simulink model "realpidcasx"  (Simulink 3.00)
settings: Solver=ode45  SolverMode=SingleTasking  StartTime=0.0  StopTime=50  FixedStep=st_size  MaxStep=st_size  RelTol=1e-5  AbsTol=1e-6
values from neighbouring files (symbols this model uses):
  Disturb = Setpoint    [mimo_MSF1DF_sim.m]    (also in mimo_MSF2DF_sim.m)
  K = 1/kpd    [imc2pseucon.m]    (also in imc2pseudo.m)
  Satlb = temp1    [cback.m]    (also in imcmenu.m = str2num(satlbs))
  Satub = temp1    [cback.m]    (also in imcmenu.m = str2num(satubs))
  Setpoint = zeros(1,n)    [mimo_MSF1DF_sim.m]    (also in mimo_MSF2DF_sim.m)
undefined symbols (not defined in the file or in its folder): conv, denCs2, K1, numCs2, Qdden, TauD, TauD1, TauI, TauI1, XdenPs, XnumPs, Xpdeadx

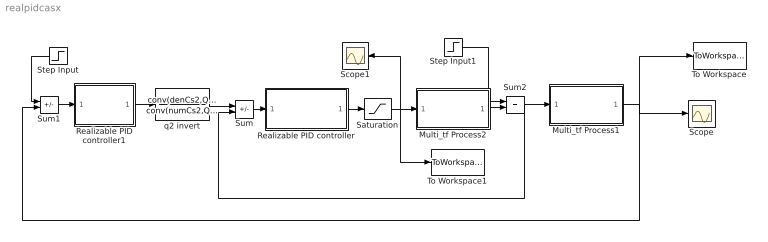
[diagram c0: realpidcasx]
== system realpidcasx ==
  Multi_tf Process1 : Subsystem
  Multi_tf Process2 : Subsystem
  Realizable PID controller : Subsystem
  Realizable PID controller1 : Subsystem
  Saturation : Saturate  UpperLimit=Satub  LowerLimit=Satlb
  Scope : Scope
  Scope1 : Scope
  Step Input : Step  Orientation=left  Time=0  Before=0  After=Setpoint  SampleTime=0
  Step Input1 : Step  Time=0  Before=0  After=Disturb  SampleTime=0
  Sum : Sum  Inputs=+-  SaturateOnIntegerOverflow=on
  Sum1 : Sum  Inputs=+-  SaturateOnIntegerOverflow=on
  Sum2 : Sum  Inputs=++  SaturateOnIntegerOverflow=on
  To Workspace : ToWorkspace  VariableName=simout  SampleTime=-1  SaveFormat=Matrix
  To Workspace1 : ToWorkspace  VariableName=effort  SampleTime=-1  SaveFormat=Matrix
  q2 invert : TransferFcn  Numerator=conv(denCs2,Qdden)  Denominator=conv(numCs2,Qdden)
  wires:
  Sum/1 -> Realizable PID controller/1(In1)
  Multi_tf Process2/1(Out1) -> Sum2/2
  Step Input1/1 -> Sum2/1
  Realizable PID controller/1(Out1) -> Saturation/1
  Saturation/1 -> To Workspace1/1, Multi_tf Process2/1(In1), Scope1/1
  Sum2/1 -> Sum/2, Multi_tf Process1/1(In1)
  Step Input/1 -> Sum1/1
  Realizable PID controller1/1(Out1) -> q2 invert/1
  Sum1/1 -> Realizable PID controller1/1(In1)
  q2 invert/1 -> Sum/1
  Multi_tf Process1/1(Out1) -> Sum1/2, To Workspace/1, Scope/1

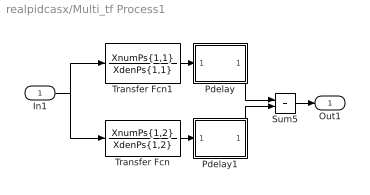
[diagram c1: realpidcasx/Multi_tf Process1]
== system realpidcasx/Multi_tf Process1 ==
  In1 : Inport  Port=1  PortWidth=-1  SampleTime=-1  DataType=auto
  Pdelay : Subsystem
  Pdelay1 : Subsystem
  Sum5 : Sum  Inputs=++  SaturateOnIntegerOverflow=on
  Transfer Fcn : TransferFcn  Numerator=XnumPs{1,2}  Denominator=XdenPs{1,2}
  Transfer Fcn1 : TransferFcn  Numerator=XnumPs{1,1}  Denominator=XdenPs{1,1}
  Out1 : Outport  Port=1  InitialOutput=0
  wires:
  Transfer Fcn1/1 -> Pdelay/1(In1)
  Transfer Fcn/1 -> Pdelay1/1(In1)
  Pdelay/1(Out1) -> Sum5/1
  In1/1 -> Transfer Fcn1/1, Transfer Fcn/1
  Sum5/1 -> Out1/1
  Pdelay1/1(Out1) -> Sum5/2

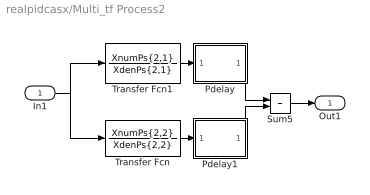
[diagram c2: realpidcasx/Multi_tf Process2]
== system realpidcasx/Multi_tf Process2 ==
  In1 : Inport  Port=1  PortWidth=-1  SampleTime=-1  DataType=auto
  Pdelay : Subsystem
  Pdelay1 : Subsystem
  Sum5 : Sum  Inputs=++  SaturateOnIntegerOverflow=on
  Transfer Fcn : TransferFcn  Numerator=XnumPs{2,2}  Denominator=XdenPs{2,2}
  Transfer Fcn1 : TransferFcn  Numerator=XnumPs{2,1}  Denominator=XdenPs{2,1}
  Out1 : Outport  Port=1  InitialOutput=0
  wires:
  Transfer Fcn1/1 -> Pdelay/1(In1)
  Transfer Fcn/1 -> Pdelay1/1(In1)
  Pdelay/1(Out1) -> Sum5/1
  Pdelay1/1(Out1) -> Sum5/2
  In1/1 -> Transfer Fcn1/1, Transfer Fcn/1
  Sum5/1 -> Out1/1

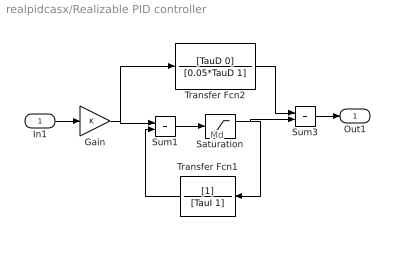
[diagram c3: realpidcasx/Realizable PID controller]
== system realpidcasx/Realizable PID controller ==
  note: Md
  In1 : Inport  Port=1  PortWidth=-1  SampleTime=-1  DataType=auto
  Gain : Gain  Gain=K  SaturateOnIntegerOverflow=on
  Saturation : Saturate  UpperLimit=Satub  LowerLimit=Satlb
  Sum1 : Sum  Inputs=++  SaturateOnIntegerOverflow=on
  Sum3 : Sum  Inputs=++  SaturateOnIntegerOverflow=on
  Transfer Fcn1 : TransferFcn  Orientation=left  Numerator=[1]  Denominator=[TauI 1]
  Transfer Fcn2 : TransferFcn  Numerator=[TauD 0]  Denominator=[0.05*TauD 1]
  Out1 : Outport  Port=1  InitialOutput=0
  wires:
  Sum1/1 -> Saturation/1
  Transfer Fcn1/1 -> Sum1/2
  Gain/1 -> Sum1/1, Transfer Fcn2/1
  Saturation/1 -> Transfer Fcn1/1, Sum3/2
  Transfer Fcn2/1 -> Sum3/1
  Sum3/1 -> Out1/1
  In1/1 -> Gain/1

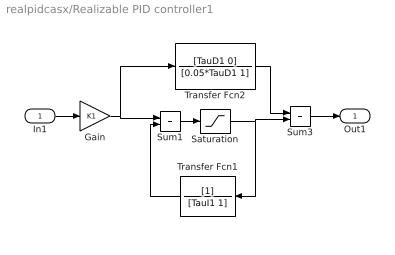
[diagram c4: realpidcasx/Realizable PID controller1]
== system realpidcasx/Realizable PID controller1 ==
  In1 : Inport  Port=1  PortWidth=-1  SampleTime=-1  DataType=auto
  Gain : Gain  Gain=K1  SaturateOnIntegerOverflow=on
  Saturation : Saturate  UpperLimit=Satub  LowerLimit=Satlb
  Sum1 : Sum  Inputs=++  SaturateOnIntegerOverflow=on
  Sum3 : Sum  Inputs=++  SaturateOnIntegerOverflow=on
  Transfer Fcn1 : TransferFcn  Orientation=left  Numerator=[1]  Denominator=[TauI1 1]
  Transfer Fcn2 : TransferFcn  Numerator=[TauD1 0]  Denominator=[0.05*TauD1 1]
  Out1 : Outport  Port=1  InitialOutput=0
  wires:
  Transfer Fcn1/1 -> Sum1/2
  Transfer Fcn2/1 -> Sum3/1
  Sum3/1 -> Out1/1
  In1/1 -> Gain/1
  Gain/1 -> Sum1/1, Transfer Fcn2/1
  Sum1/1 -> Saturation/1
  Saturation/1 -> Sum3/2, Transfer Fcn1/1

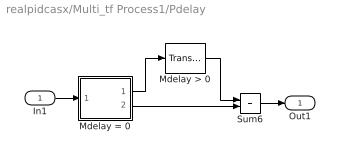
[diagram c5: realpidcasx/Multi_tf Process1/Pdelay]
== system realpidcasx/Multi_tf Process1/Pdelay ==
  In1 : Inport  Port=1  PortWidth=-1  SampleTime=-1  DataType=auto
  Mdelay > 0 : TransportDelay  DelayTime=Xpdeadx{1,1}  InitialInput=0  BufferSize=1024
  Mdelay = 0 : Subsystem  Description=pass input signal through out1 if condition is true.
  Sum6 : Sum  Inputs=++  SaturateOnIntegerOverflow=on
  Out1 : Outport  Port=1
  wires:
  Mdelay = 0/1(Out2) -> Mdelay > 0/1
  Mdelay > 0/1 -> Sum6/1
  Mdelay = 0/2(Out1) -> Sum6/2
  In1/1 -> Mdelay = 0/1(In)
  Sum6/1 -> Out1/1

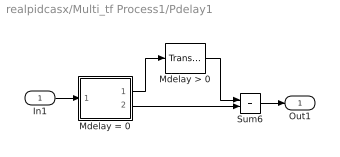
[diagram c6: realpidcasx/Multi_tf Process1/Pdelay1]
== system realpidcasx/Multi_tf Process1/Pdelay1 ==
  In1 : Inport  Port=1  PortWidth=-1  SampleTime=-1  DataType=auto
  Mdelay > 0 : TransportDelay  DelayTime=Xpdeadx{1,2}  InitialInput=0  BufferSize=1024
  Mdelay = 0 : Subsystem  Description=pass input signal through out1 if condition is true.
  Sum6 : Sum  Inputs=++  SaturateOnIntegerOverflow=on
  Out1 : Outport  Port=1
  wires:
  Mdelay = 0/1(Out2) -> Mdelay > 0/1
  Mdelay > 0/1 -> Sum6/1
  Mdelay = 0/2(Out1) -> Sum6/2
  In1/1 -> Mdelay = 0/1(In)
  Sum6/1 -> Out1/1

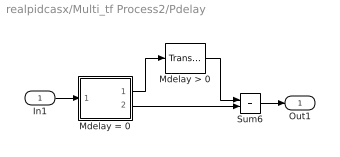
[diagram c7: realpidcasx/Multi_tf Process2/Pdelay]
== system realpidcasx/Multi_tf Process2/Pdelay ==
  In1 : Inport  Port=1  PortWidth=-1  SampleTime=-1  DataType=auto
  Mdelay > 0 : TransportDelay  DelayTime=Xpdeadx{2,1}  InitialInput=0  BufferSize=1024
  Mdelay = 0 : Subsystem  Description=pass input signal through out1 if condition is true.
  Sum6 : Sum  Inputs=++  SaturateOnIntegerOverflow=on
  Out1 : Outport  Port=1
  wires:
  Mdelay = 0/1(Out2) -> Mdelay > 0/1
  Mdelay > 0/1 -> Sum6/1
  Mdelay = 0/2(Out1) -> Sum6/2
  In1/1 -> Mdelay = 0/1(In)
  Sum6/1 -> Out1/1

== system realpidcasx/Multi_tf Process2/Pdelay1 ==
  In1 : Inport  Port=1  PortWidth=-1  SampleTime=-1  DataType=auto
  Mdelay > 0 : TransportDelay  DelayTime=Xpdeadx{2,2}  InitialInput=0  BufferSize=1024
  Mdelay = 0 : Subsystem  Description=pass input signal through out1 if condition is true.
  Sum6 : Sum  Inputs=++  SaturateOnIntegerOverflow=on
  Out1 : Outport  Port=1
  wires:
  Mdelay = 0/1(Out2) -> Mdelay > 0/1
  Mdelay > 0/1 -> Sum6/1
  Mdelay = 0/2(Out1) -> Sum6/2
  In1/1 -> Mdelay = 0/1(In)
  Sum6/1 -> Out1/1

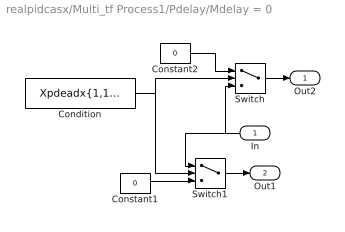
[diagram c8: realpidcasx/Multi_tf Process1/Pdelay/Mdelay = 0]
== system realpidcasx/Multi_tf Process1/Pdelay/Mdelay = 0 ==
  In : Inport  Orientation=left  Port=1  PortWidth=-1  SampleTime=-1  DataType=auto
  Condition : Constant  Value=Xpdeadx{1,1}<=3*eps
  Constant1 : Constant  Value=0
  Constant2 : Constant  Value=0
  Switch : Switch  Threshold=1
  Switch1 : Switch  Threshold=1
  Out2 : Outport  Port=1  InitialOutput=0
  Out1 : Outport  Port=2  InitialOutput=0
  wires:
  In/1 -> Switch/3, Switch1/1
  Condition/1 -> Switch1/2, Switch/2
  Constant1/1 -> Switch1/3
  Constant2/1 -> Switch/1
  Switch/1 -> Out2/1
  Switch1/1 -> Out1/1

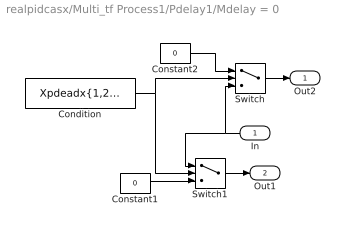
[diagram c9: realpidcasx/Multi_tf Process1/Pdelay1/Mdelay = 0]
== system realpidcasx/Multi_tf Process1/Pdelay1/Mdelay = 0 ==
  In : Inport  Orientation=left  Port=1  PortWidth=-1  SampleTime=-1  DataType=auto
  Condition : Constant  Value=Xpdeadx{1,2}<=3*eps
  Constant1 : Constant  Value=0
  Constant2 : Constant  Value=0
  Switch : Switch  Threshold=1
  Switch1 : Switch  Threshold=1
  Out2 : Outport  Port=1  InitialOutput=0
  Out1 : Outport  Port=2  InitialOutput=0
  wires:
  In/1 -> Switch/3, Switch1/1
  Condition/1 -> Switch1/2, Switch/2
  Constant1/1 -> Switch1/3
  Constant2/1 -> Switch/1
  Switch/1 -> Out2/1
  Switch1/1 -> Out1/1

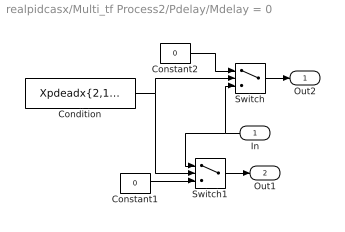
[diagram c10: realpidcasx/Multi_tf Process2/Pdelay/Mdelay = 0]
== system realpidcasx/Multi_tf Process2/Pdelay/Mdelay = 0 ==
  In : Inport  Orientation=left  Port=1  PortWidth=-1  SampleTime=-1  DataType=auto
  Condition : Constant  Value=Xpdeadx{2,1}<=3*eps
  Constant1 : Constant  Value=0
  Constant2 : Constant  Value=0
  Switch : Switch  Threshold=1
  Switch1 : Switch  Threshold=1
  Out2 : Outport  Port=1  InitialOutput=0
  Out1 : Outport  Port=2  InitialOutput=0
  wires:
  In/1 -> Switch/3, Switch1/1
  Condition/1 -> Switch1/2, Switch/2
  Constant1/1 -> Switch1/3
  Constant2/1 -> Switch/1
  Switch/1 -> Out2/1
  Switch1/1 -> Out1/1

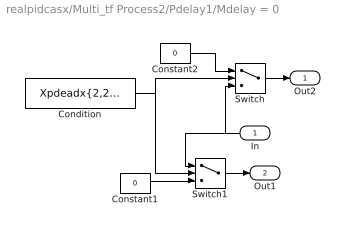
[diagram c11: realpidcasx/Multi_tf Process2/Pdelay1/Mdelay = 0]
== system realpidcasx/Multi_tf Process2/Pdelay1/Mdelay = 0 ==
  In : Inport  Orientation=left  Port=1  PortWidth=-1  SampleTime=-1  DataType=auto
  Condition : Constant  Value=Xpdeadx{2,2}<=3*eps
  Constant1 : Constant  Value=0
  Constant2 : Constant  Value=0
  Switch : Switch  Threshold=1
  Switch1 : Switch  Threshold=1
  Out2 : Outport  Port=1  InitialOutput=0
  Out1 : Outport  Port=2  InitialOutput=0
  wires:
  In/1 -> Switch/3, Switch1/1
  Condition/1 -> Switch1/2, Switch/2
  Constant1/1 -> Switch1/3
  Constant2/1 -> Switch/1
  Switch/1 -> Out2/1
  Switch1/1 -> Out1/1
